//{{V2}}
ORGANIZATION_BLOCK OB1
TITLE= "Main Program Sweep (Cycle)"


AUTHOR:nb
FAMILY:nb
NAME:nb
VERSION:00.01


VAR_TEMP
       OB1_EV_CLASS:BYTE //Bits 0-3 = 1 (Coming event), Bits 4-7 = 1 (Event class 1)
       OB1_SCAN_1:BYTE //1 (Cold restart scan 1 of OB 1), 3 (Scan 2-n of OB 1)
       OB1_PRIORITY:BYTE //Priority of OB Execution
       OB1_OB_NUMBR:BYTE //1 (Organization block 1, OB1)
       OB1_RESERVED_1:BYTE //Reserved for system
       OB1_RESERVED_2:BYTE //Reserved for system
       OB1_PREV_CYCLE:INT //Cycle time of previous OB1 scan (milliseconds)
       OB1_MIN_CYCLE:INT //Minimum cycle time of OB1 (milliseconds)
       OB1_MAX_CYCLE:INT //Maximum cycle time of OB1 (milliseconds)
       OB1_DATE_TIME:DATE_AND_TIME //Date and time OB1 started
       Done:BOOL
       Error:BOOL
       ErrorNum:DINT
       NodeId:BYTE
       xDInt:DINT
END_VAR
BEGIN

NETWORK
TITLE=
//{{a}}

// Initialisation
       L    4
       T    #NodeId

       U    E         0.6
       =    A         0.6

       CALL FB91,DB91
         Write:=E0.0                     // Input 0
         NodeID:=#NodeId
         Done:=#Done
         Err:=#Error
         ErrNo:=#ErrorNum

       CALL FB99,DB99
         Write:=E0.0                     // Input 0
         NodeID:=#NodeId
         Mode:=B#16#FE                   // Velocity Mode
         Done:=#Done
         Err:=#Error
         ErrNo:=#ErrorNum

       CALL FB98,DB98
         Write:=E0.6                     // Input 1
         NodeID:=#NodeId
         Done:=#Done
         Err:=#Error
         ErrNo:=#ErrorNum

       CALL FB97,DB97
         Write:=E0.7                     // Input 2
         NodeID:=#NodeId
         Done:=#Done
         Err:=#Error
         ErrNo:=#ErrorNum

// Programm Start

       L    15
       T    #xDInt

       CALL FB112,DB112
         Write:=E0.1
         NodeID:=#NodeId
         VelocityMust:=#xDInt
         Done:=#Done
         Err:=#Error
         ErrNo:=#ErrorNum

       CALL FB53,DB53
         Read:=E0.2
         NodeID:=#NodeId
         Done:=#Done
         Err:=#Error
         ErrNo:=#ErrorNum
         PositionIs:=MD200
END_ORGANIZATION_BLOCK
